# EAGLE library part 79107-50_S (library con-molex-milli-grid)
RECEPTACAL
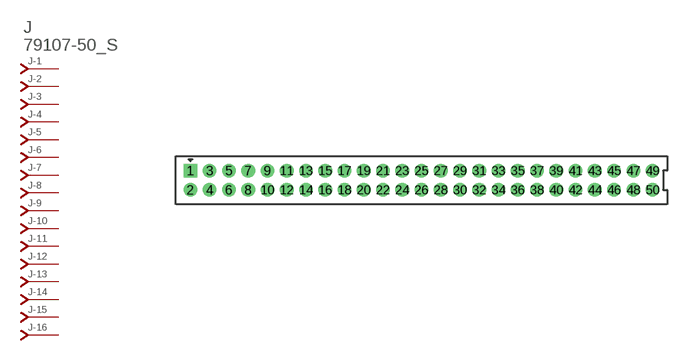
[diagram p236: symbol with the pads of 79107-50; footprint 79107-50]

Designator prefix J; gates -1=J-NV -2=J-N -3=J-N -4=J-N -5=J-N -6=J-N -7=J-N -8=J-N -9=J-N -10=J-N -11=J-N -12=J-N -13=J-N -14=J-N -15=J-N -16=J-N -17=J-N -18=J-N -19=J-N -20=J-N -21=J-N -22=J-N -23=J-N -24=J-N -25=J-N -26=J-N -27=J-N -28=J-N -29=J-N -30=J-N -31=J-N -32=J-N -33=J-N -34=J-N -35=J-N -36=J-N -37=J-N -38=J-N -39=J-N -40=J-N -41=J-N -42=J-N -43=J-N -44=J-N -45=J-N -46=J-N -47=J-N -48=J-N -49=J-N -50=J-N

## 79107-50_S  [79107-50]
1  -1:J  pas
2  -2:J  pas
3  -3:J  pas
4  -4:J  pas
5  -5:J  pas
6  -6:J  pas
7  -7:J  pas
8  -8:J  pas
9  -9:J  pas
10  -10:J  pas
11  -11:J  pas
12  -12:J  pas
13  -13:J  pas
14  -14:J  pas
15  -15:J  pas
16  -16:J  pas
17  -17:J  pas
18  -18:J  pas
19  -19:J  pas
20  -20:J  pas
21  -21:J  pas
22  -22:J  pas
23  -23:J  pas
24  -24:J  pas
25  -25:J  pas
26  -26:J  pas
27  -27:J  pas
28  -28:J  pas
29  -29:J  pas
30  -30:J  pas
31  -31:J  pas
32  -32:J  pas
33  -33:J  pas
34  -34:J  pas
35  -35:J  pas
36  -36:J  pas
37  -37:J  pas
38  -38:J  pas
39  -39:J  pas
40  -40:J  pas
41  -41:J  pas
42  -42:J  pas
43  -43:J  pas
44  -44:J  pas
45  -45:J  pas
46  -46:J  pas
47  -47:J  pas
48  -48:J  pas
49  -49:J  pas
50  -50:J  pas

## Footprint 79107-50 (pad centres in mm)
RECEPTACAL Dual Row, Vertical, Through-Hole
drill 0.914 square: 1 -24,1
drill 0.914: 2 -24,-1; 3 -22,1; 4 -22,-1; 5 -20,1; 6 -20,-1; 7 -18,1; 8 -18,-1; 9 -16,1; 10 -16,-1; 11 -14,1; 12 -14,-1; 13 -12,1; 14 -12,-1; 15 -10,1; 16 -10,-1; 17 -8,1; 18 -8,-1; 19 -6,1; 20 -6,-1; 21 -4,1; 22 -4,-1; 23 -2,1; 24 -2,-1; 25 0,1; 26 0,-1; 27 2,1; 28 2,-1; 29 4,1; 30 4,-1; 31 6,1; 32 6,-1; 33 8,1; 34 8,-1; 35 10,1; 36 10,-1; 37 12,1; 38 12,-1; 39 14,1; 40 14,-1; 41 16,1; 42 16,-1; 43 18,1; 44 18,-1; 45 20,1; 46 20,-1; 47 22,1; 48 22,-1; 49 24,1; 50 24,-1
